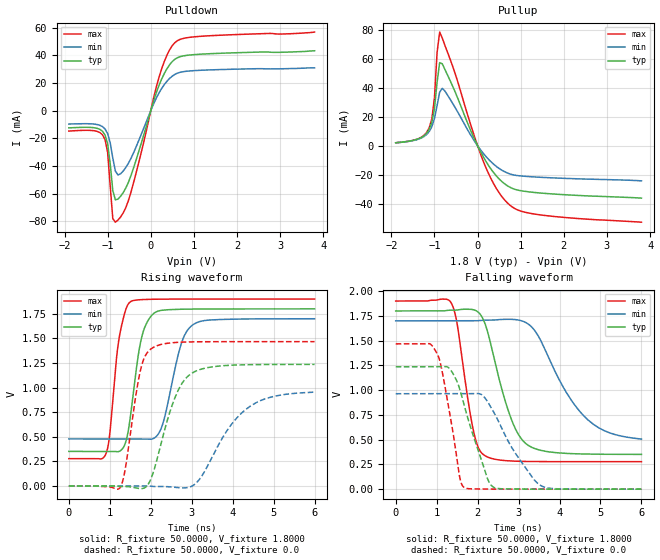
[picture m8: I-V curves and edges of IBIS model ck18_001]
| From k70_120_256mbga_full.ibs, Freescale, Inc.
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|   Model ck18_001
[Model]  ck18_001
Model_type Output
Polarity   Non-Inverting
Enable   Active-High
Vmeas =  0.9000V
Cref =   5.0000pF
Rref =   50.0000
C_comp   2.8000pF   2.5000pF   3.3000pF
[Temperature Range]   25.0000   0.1250k   -40.0000
[Voltage Range]   1.8000V   1.7000V   1.9000V
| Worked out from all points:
|   slope of the pulldown table from 0 to 0.27 V, typ, clamps not added: 11.2 ohm
|   slope of the pullup table from 0 to 0.27 V, typ, clamps not added: 18.8 ohm
|   rising waveform, R_fixture 50.0000, V_fixture 1.8000: 20-80 % time 296ps typ, 400ps min, 242ps max; typ from 0.351 V to 1.8 V
|   rising waveform, R_fixture 50.0000, V_fixture 0.0: 20-80 % time 551ps typ, 906ps min, 324ps max; typ from 0 V to 1.24 V
|   falling waveform, R_fixture 50.0000, V_fixture 1.8000: 20-80 % time 595ps typ, 994ps min, 356ps max; typ from 1.8 V to 0.351 V
|   falling waveform, R_fixture 50.0000, V_fixture 0.0: 20-80 % time 552ps typ, 806ps min, 357ps max; typ from 1.24 V to 0 V
[Pulldown]
|Voltage   I(typ)   I(min)   I(max)
-1.9V     -12.39mA   -9.607mA   -14.7mA
-1.24V    -12.76mA   -10.02mA   -14.96mA
-1.06V    -17.57mA   -13.18mA   -20.87mA
-1V       -23.84mA   -16.51mA   -30.07mA
-880mV    -57.69mA   -34.18mA   -77.94mA
-820mV    -64.38mA   -43.64mA   -80.54mA
-700mV    -61.85mA   -45.6mA    -76.8mA
-520mV    -51.88mA   -38.08mA   -65.12mA
200mV     18.95mA    13.28mA    25.03mA
380mV     30.52mA    21.42mA    40.4mA
560mV     37.18mA    26.25mA    49.21mA
3.8V      43.3mA     31mA       56.8mA
[Pullup]
|Voltage   I(typ)   I(min)   I(max)
-1.9V     2.1mA      2.1mA      2.1mA
-1.36V    4.99mA     4.72mA     5.12mA
-1.12V    11.5mA     9.96mA     12.59mA
-1.06V    16.35mA    13.28mA    18.88mA
-1V       25.93mA    18.84mA    33.41mA
-940mV    43.83mA    27.8mA     64.36mA
-880mV    57.43mA    37.06mA    78.47mA
-760mV    52.81mA    37.83mA    69.41mA
140mV     -8.034mA   -5.522mA   -11.29mA
680mV     -27.38mA   -18.63mA   -39.1mA
1.4V      -32.43mA   -21.63mA   -47.46mA
3.8V      -36.11mA   -24.19mA   -52.72mA
[Ramp]
| variable   typ   min   max
dV/dt_r  0.7414/0.5513n   0.5722/0.9061n   0.8803/0.3239n
dV/dt_f  0.8693/0.5948n   0.7164/0.9941n   0.9734/0.3556n
R_load = 50.0000
[Rising Waveform]
R_fixture= 50.0000
V_fixture= 1.8000
V_fixture_min= 1.7000
V_fixture_max= 1.9000
|time   V(typ)   V(min)   V(max)
0s        351mV      477.7mV    277.7mV
913.1ps   351mV      477.7mV    333.6mV
1.225ns   350.5mV    477.7mV    1.495V
1.502ns   699.2mV    477.7mV    1.872V
1.78ns    1.513V     477.9mV    1.894V
2.105ns   1.764V     491.9mV    1.898V
2.311ns   1.788V     653.7mV    1.899V
2.76ns    1.797V     1.464V     1.9V
3.034ns   1.798V     1.64V      1.9V
6ns       1.8V       1.7V       1.9V
[Rising Waveform]
R_fixture= 50.0000
V_fixture= 0.0
|time   V(typ)   V(min)   V(max)
0s        2.964nV    322.7nV    772.1pV
1.261ns   -6.299mV   681nV      -10.55mV
1.389ns   -5.903mV   554.8nV    198.7mV
1.747ns   -26.77mV   30.35uV    1.173V
2.035ns   103.7mV    -4.434mV   1.402V
2.553ns   856mV      -12.58mV   1.457V
2.975ns   1.138V     -7.695mV   1.465V
4.332ns   1.232V     781.2mV    1.467V
4.912ns   1.235V     901.1mV    1.467V
6ns       1.236V     953.7mV    1.467V
[Falling Waveform]
R_fixture= 50.0000
V_fixture= 1.8000
V_fixture_min= 1.7000
V_fixture_max= 1.9000
|time   V(typ)   V(min)   V(max)
0s        1.8V       1.7V       1.9V
1.368ns   1.807V     1.7V       1.872V
1.51ns    1.81V      1.7V       1.647V
1.901ns   1.812V     1.7V       584.1mV
2.178ns   1.674V     1.706V     338.2mV
2.738ns   805.9mV    1.716V     286.4mV
3.156ns   467.3mV    1.687V     280mV
3.452ns   402mV      1.567V     278.6mV
4.59ns    355.2mV    741.3mV    277.7mV
6ns       351.2mV    506mV      277.7mV
[Falling Waveform]
R_fixture= 50.0000
V_fixture= 0.0
|time   V(typ)   V(min)   V(max)
0s        1.236V     963.8mV    1.467V
826ps     1.236V     963.8mV    1.469V
1.02ns    1.236V     963.8mV    1.363V
1.359ns   1.194V     963.8mV    674.1mV
1.56ns    1.016V     963.8mV    128mV
1.674ns   845.7mV    963.7mV    16.19mV
2.093ns   296mV      955.2mV    1.426mV
2.395ns   18.39mV    777.2mV    561.2uV
3.551ns   386uV      34.62mV    14.83uV
6ns       1.863uV    125.7uV    36.79nV
